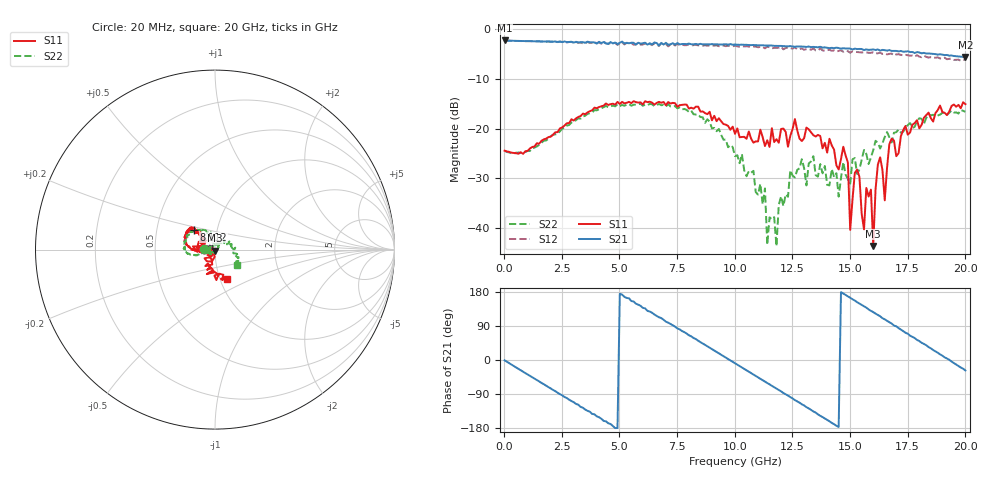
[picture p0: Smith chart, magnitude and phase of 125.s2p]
!Agilent Technologies,N5230A,US43500223,A.07.50.48
!Agilent N5230A: A.07.50.48
!Date: Tuesday, November 17, 2015 13:39:36
!Correction: S11(Full 2 Port(1,2))
!S21(Full 2 Port(1,2))
!S12(Full 2 Port(1,2))
!S22(Full 2 Port(1,2))
!S2P File: Measurements: S11, S21, S12, S22:
# Hz S  dB  R 50
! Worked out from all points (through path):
!   201 points, 20 MHz to 20 GHz, reference 50 ohm
!   highest |S21| = -2.33 dB at 20 MHz (marker M1); lowest = -5.7 dB at 20 GHz (marker M2)
!   group delay of S21, straight-line fit = 103 ps
!   lowest |S11| = -43.5 dB at 16 GHz (marker M3), VSWR 1.01, Z = 49.9 - j0.663 ohm
!   |S11| at or under -10 dB: start of sweep to end of sweep
!   |S22| runs from -43.6 to -15.0 dB; largest |S21 - S12| = 0.083
!   S11 on the Smith chart (normalised r, x): 20 MHz: 0.89, +0.00; 8.112 GHz: 0.77, +0.18; 20 GHz: 1.08, -0.36
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2e7  -24.44 179.1  -2.33 -0.8  -2.33 -0.9  -24.46 178.9
1.9181e9  -21.72 -173.0  -2.51 -71.5  -2.56 -72.6  -22.04 -164.9
3.4166e9  -17.00 176.0  -2.67 -126.0  -2.93 -127.2  -17.58 -167.6
5.1149e9  -14.65 154.2  -2.56 172.5  -2.71 169.7  -15.28 176.0
6.7133e9  -14.65 142.5  -3.35 112.7  -3.44 110.6  -15.06 153.5
8.1119e9  -15.82 136.3  -3.09 62.4  -3.40 58.8  -16.40 132.2
1.001e10  -21.05 137.3  -3.16 -8.3  -3.38 -11.9  -25.53 83.2
1.18082e10  -22.14 150.9  -3.42 -75.6  -3.84 -79.6  -43.58 -47.9
1.24076e10  -21.47 -177.5  -3.47 -98.0  -3.87 -103.2  -28.37 -140.1
1.34066e10  -21.32 -176.4  -3.62 -135.8  -3.95 -139.2  -25.53 -170.8
1.45055e10  -28.20 -169.1  -3.84 -176.6  -4.43 179.8  -33.63 115.3
1.47053e10  -23.65 -161.3  -3.90 175.4  -4.60 171.9  -26.71 108.6
1.49051e10  -26.81 159.3  -3.93 167.8  -4.50 163.6  -30.12 95.9
1.5005e10  -40.32 154.2  -3.97 164.3  -4.80 160.4  -31.07 74.5
1.52048e10  -28.90 -129.3  -3.98 156.9  -4.61 152.0  -25.92 75.3
1.56044e10  -40.21 -138.2  -4.26 142.0  -4.72 138.3  -24.29 53.2
1.59041e10  -32.25 -163.4  -4.19 129.6  -4.82 127.1  -25.78 45.1
1.6004e10  -43.53 -94.5  -4.13 126.4  -4.71 122.2  -24.34 29.7
1.62038e10  -27.25 -117.5  -4.13 118.8  -4.91 114.6  -22.83 45.8
1.65035e10  -34.39 -113.3  -4.28 107.4  -4.95 103.4  -21.69 24.3
1.67033e10  -23.11 -104.7  -4.26 99.7  -5.03 95.7  -21.73 29.7
2e10  -15.11 -68.2  -5.65 -27.6  -6.19 -33.4  -16.64 -34.5
